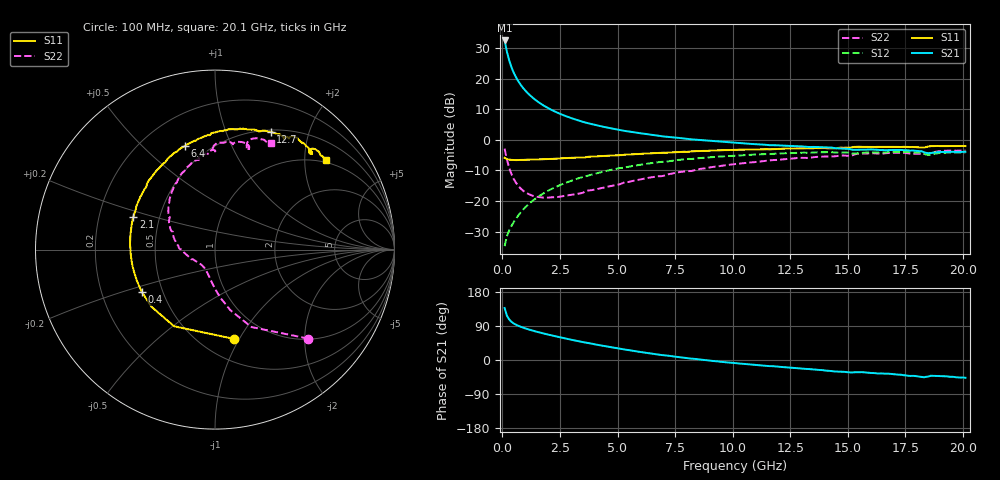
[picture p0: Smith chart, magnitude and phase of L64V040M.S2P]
!  Infineon Technologies AG
! BFR380L3 , PF131585-7, No.6, Th 09.10.01, soldered on pcb-board, measured with PP GSG850
!  Vce=4.0 V,  Ic=40.0 mA
! Common Emitter S-Parameters:  15. November 2001
#  GHz  S  MA  R  50
! f  S11  S21  S12  S22
! GHz  Mag  Ang  Mag  Ang  Mag  Ang  Mag  Ang
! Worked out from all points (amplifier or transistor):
!   201 points, 100 MHz to 20.1 GHz, reference 50 ohm
!   highest |S21| = 32.5 dB at 100 MHz (marker M1)
!   |S21| within 3 dB of that: start of sweep to 181.5 MHz
!   unconditionally stable (mu >= 1): 1.096 GHz to 4.291 GHz
!   at 3.4 GHz: K = 1.02, MAG = 8.5 dB, |S12| = -12.3 dB
!   at 10.1 GHz: K = 0.95, MSG = 2.1 dB, |S12| = -5.1 dB
!   at 20.1 GHz: K = 0.98, MSG = 0.1 dB, |S12| = -4.1 dB
!   S11 on the Smith chart (normalised r, x): 100 MHz: 0.71, -0.95; 400 MHz: 0.38, -0.23; 2.1 GHz: 0.35, +0.17; 6.4 GHz: 0.38, +0.68; 12.7 GHz: 0.52, +1.45; 20.1 GHz: 0.95, +2.52
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0.1  0.5088 -77.9  42.28 137.2  0.0183 63.4  0.7182 -43.6
0.2  0.4842 -118.1  27.68 116.8  0.02659 57.6  0.4771 -64.8
0.3  0.4762 -138.1  19.86 106.9  0.03317 58.4  0.3481 -75.8
0.4  0.4711 -150.1  15.35 100.7  0.03927 60.4  0.2746 -83.0
0.5  0.4687 -158.1  12.46 96.3  0.04562 62.7  0.2285 -88.5
0.6  0.4677 -164.0  10.48 92.9  0.05213 64.3  0.1978 -93.0
0.7  0.4688 -168.9  9.039 90.0  0.05858 65.4  0.176 -97.0
0.9  0.47 -176.0  7.087 85.4  0.07227 67.0  0.148 -103.8
1.1  0.4727 178.3  5.841 81.4  0.086 67.6  0.1326 -110.1
1.4  0.4775 171.4  4.625 76.1  0.1067 67.6  0.1198 -118.1
1.7  0.4821 165.5  3.838 71.4  0.1274 66.8  0.1149 -125.3
2.1  0.4888 158.4  3.142 65.5  0.1549 65.2  0.1149 -133.7
2.7  0.5025 149.1  2.494 57.3  0.1953 61.9  0.1214 -145.5
3.5  0.518 137.9  1.973 47.2  0.2484 56.9  0.1368 -157.0
4.9  0.5593 121.4  1.501 31.7  0.3336 47.4  0.1816 -178.4
6.4  0.6014 106.1  1.222 17.5  0.4144 37.0  0.2423 162.8
6.8  0.6124 102.3  1.168 14.1  0.4333 34.0  0.2546 157.9
10.1  0.6886 78.3  0.8971 -8.2  0.5538 12.3  0.4022 126.7
12.7  0.7251 64.6  0.7897 -21.3  0.6131 -3.6  0.5008 105.0
13.5  0.73 60.9  0.7681 -25.0  0.6211 -8.3  0.5192 99.6
16.8  0.769 48.4  0.6864 -36.3  0.6296 -24.4  0.6119 78.5
20.1  0.792 38.9  0.6395 -46.9  0.624 -38.2  0.6711 62.2
